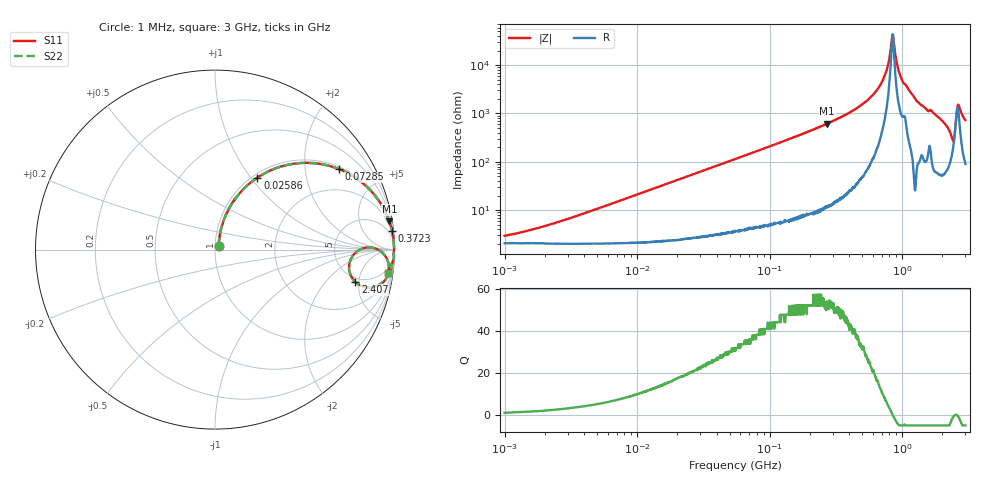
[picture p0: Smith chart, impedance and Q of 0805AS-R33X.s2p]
!s-Parameter Generated by FASTRON Sdn. Bhd.
!FASTRON P/N : 0805AS-R33X
!Keysight Technologies: E4991B_MY54100416_A.01.15
!Date: Mon Jun 15 12:54:15 2026
!Version  :Rev01  Mon Jun 15 12:54:15 2026
!Data & Calibration Information:
!Freq  S11  S21  S12  S22
!PortZ  Port1:50+j0  Port2:50+j0
!When reading reference impedance value at option line is always used.
! Remarks : This data is being provided solely for informational purposes.
# Hz S dB R 50
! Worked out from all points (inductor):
!   1601 points, 1 MHz to 3 GHz, reference 50 ohm
!   read as one part in series: L = 335 nH near 2.889 MHz
!   highest Q = 53.5 at 271.6 MHz (marker M1), where L = 360 nH
!   self-resonance near 845.9 MHz
!   S11 on the Smith chart (normalised r, x): 1 MHz: 1.04, +0.04; 25.86 MHz: 1.05, +1.08; 72.85 MHz: 1.09, +3.03; 372.3 MHz: 1, +19; 2.407 GHz: 4.44, -4.48; 3 GHz: 3, -15
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1000000  -30.80 44.3  -0.18 -1.2  -0.18 -1.2  -30.80 44.3
3804036  -21.90 71.4  -0.20 -4.5  -0.20 -4.5  -21.90 71.4
1.447069e7  -10.90 69.2  -0.56 -16.5  -0.56 -16.5  -10.90 69.2
2.585714e7  -6.63 59.5  -1.29 -27.7  -1.29 -27.7  -6.63 59.5
5.504702e7  -2.60 40.3  -3.77 -47.8  -3.77 -47.8  -2.60 40.3
7.285059e7  -1.68 32.9  -5.29 -55.5  -5.29 -55.5  -1.68 32.9
2.083556e8  -0.24 12.4  -13.40 -76.5  -13.40 -76.5  -0.24 12.4
2.716345e8  -0.14 9.2  -15.90 -79.7  -15.90 -79.7  -0.14 9.2
3.72303e8  -0.07 6.1  -19.50 -82.7  -19.50 -82.7  -0.07 6.1
6.264832e8  -0.02 2.1  -28.90 -84.8  -28.90 -84.8  -0.02 2.1
7.243229e8  -0.02 1.1  -34.50 -82.7  -34.50 -82.7  -0.02 1.1
7.925923e8  -0.02 0.5  -41.40 -74.9  -41.40 -74.9  -0.02 0.5
8.291033e8  -0.02 0.2  -49.10 -51.1  -49.10 -51.1  -0.02 0.2
8.543737e8  -0.02 -0.0  -52.30 20.7  -52.30 20.7  -0.02 -0.0
9.395906e8  -0.02 -0.7  -37.80 77.2  -37.80 77.2  -0.02 -0.7
1.023018e9  -0.04 -1.3  -32.70 77.1  -32.70 77.1  -0.04 -1.3
1.327057e9  -0.04 -3.4  -24.60 83.5  -24.60 83.5  -0.04 -3.4
2.050964e9  -0.20 -8.5  -16.60 76.8  -16.60 76.8  -0.20 -8.5
2.407135e9  -1.92 -13.0  -11.00 39.4  -11.00 39.4  -1.92 -13.0
2.543347e9  -1.18 0.7  -17.90 -5.1  -17.90 -5.1  -1.18 0.7
2.660507e9  -0.41 -2.6  -23.90 42.5  -23.90 42.5  -0.41 -2.6
3e9  -0.22 -7.6  -17.50 75.3  -17.50 75.3  -0.22 -7.6
